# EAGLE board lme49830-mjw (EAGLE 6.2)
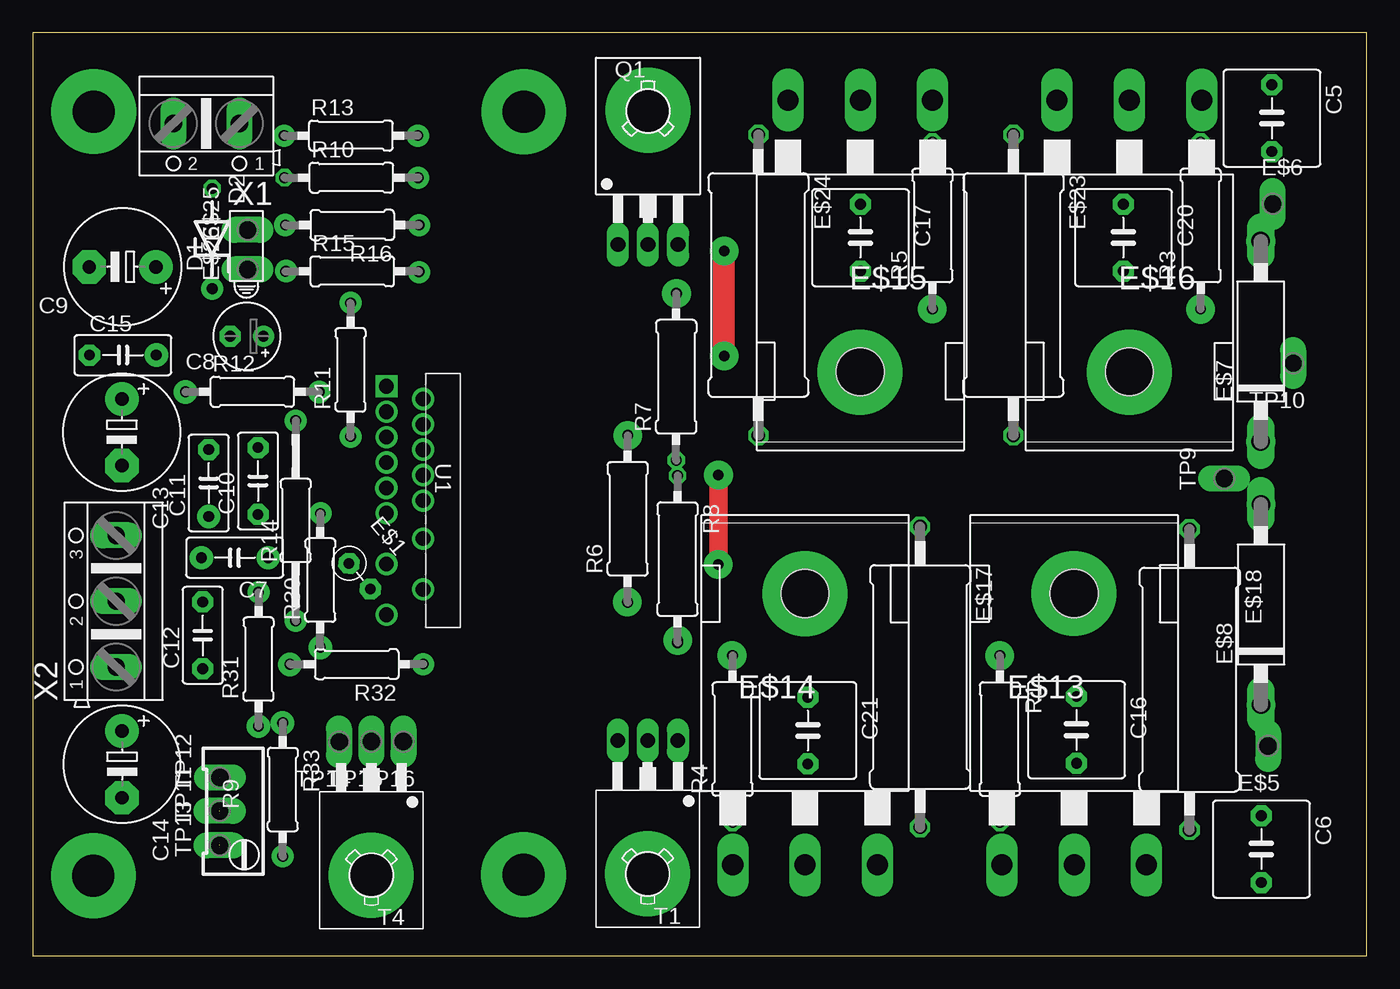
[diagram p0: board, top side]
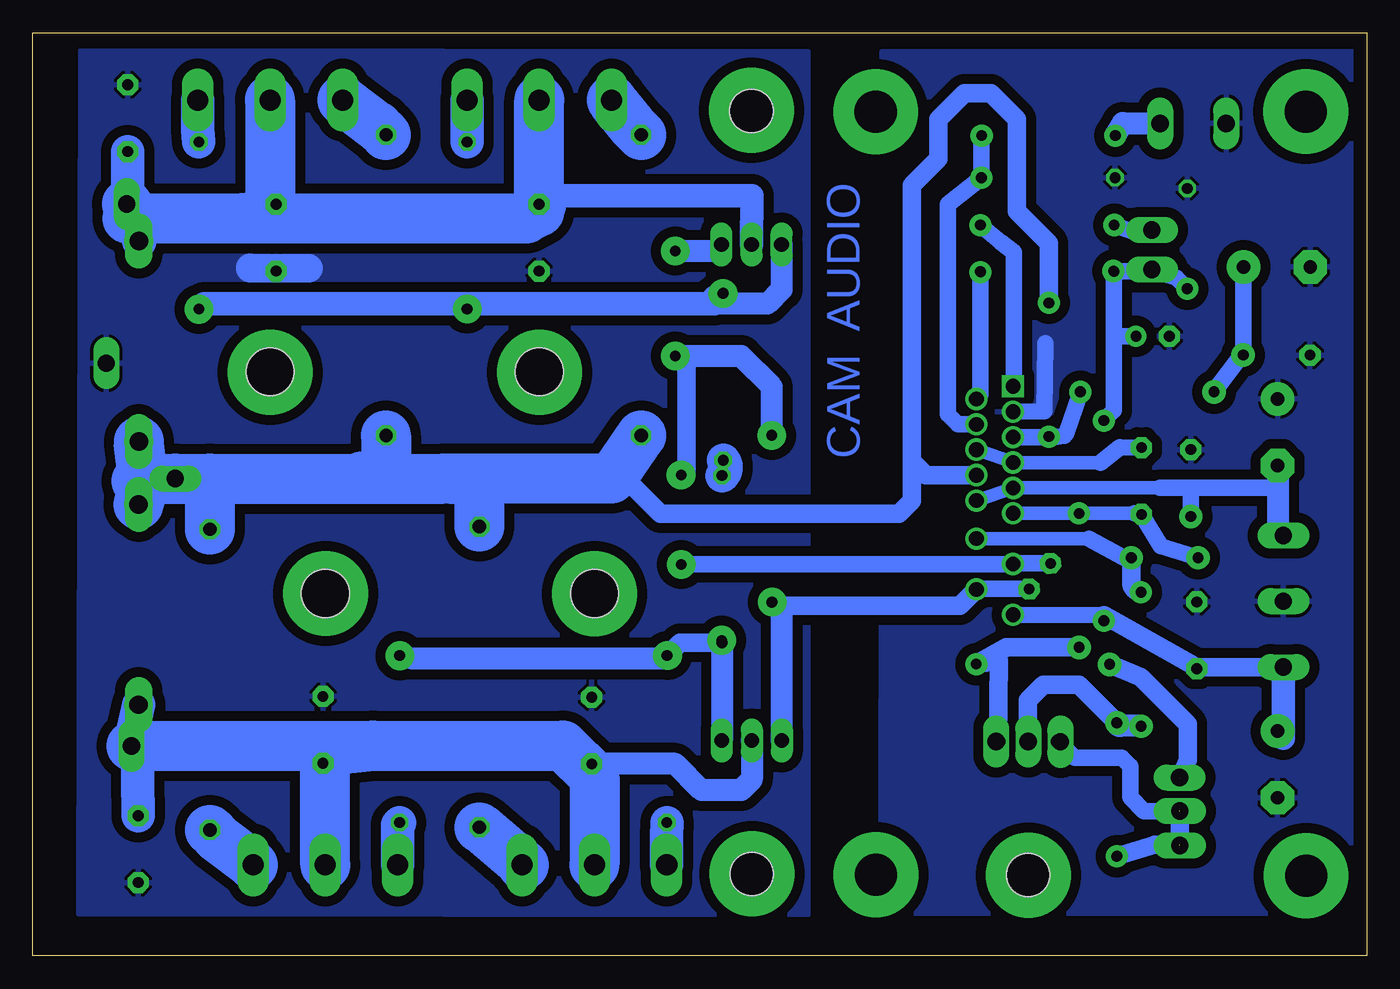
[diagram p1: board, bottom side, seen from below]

Size 101.46 x 70.17 mm. Coordinates in mm from the lower left corner, seen from the top.
Outline: 0,0 101.46,0 101.46,70.17 0,70.17 0,0
Copper layers (1*16): Top 0.035mm / dielectric 1.5mm / Bottom 0.035mm
Design rules: minimum track width 10mil, minimum drill 24mil, track to track 30mil, track to pad 30mil, pad to pad 30mil, via to via 30mil, smd to smd 30mil, copper to edge 40mil, drill to drill 8mil, minimum pad ring 10mil, minimum via ring 8mil, stop-mask expansion 4mil, vias tented up to drill 0mil, thermal gap 10mil
vRestrict: area 32.5,1.9 to 43.5,68.9

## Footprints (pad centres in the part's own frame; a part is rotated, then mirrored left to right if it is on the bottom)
C5B7.2 = drill 0.813 pad 1.6 octagon: 1 -2.54,0; 2 2.54,0
C5B3 = drill 0.813 pad 1.6 octagon: 1 -2.54,0; 2 2.54,0
E2,5-5 = drill 0.813 pad 1.6: + -1.27,0 | drill 0.813 pad 1.6 octagon: - 1.27,0
E5-8,5 = drill 1.016 pad 2.54: + -2.54,0 | drill 1.016 pad 2.54 octagon: - 2.54,0
ZDIO-7.5 = drill 0.813 octagon: A 3.81,0; C -3.81,0
HLMP6 = drill 0.813 long: A -1.27,0; K 1.27,0
RS-2,5 = drill 0.813 pad 1.6 octagon: 1 -1.27,0; 2 1.27,0
P1-13Y = drill 1.321 pad 1.905 long: TP 0,0
C1702E15 = drill 1.397 long: A 7.62,0; C -7.62,0
TO-247AD-H = drill 1.6 long: D 0,-20.65; G -5.5,-20.65; S 5.5,-20.65 | hole 3.65: 0,0
P0817/22 = drill 1.016 octagon: 1 -11.43,0; 2 11.43,0
TO126 = drill 1.118 long: 1 -2.286,-5.08; 2 0,-5.08; 3 2.286,-5.08 | hole 3.302: 0,5.08
0309/12 = drill 0.813 octagon: 1 -6.35,0; 2 6.35,0
RTRIM64W = drill 0.61: 1 1.27,-2.54; 2 1.27,0; 3 1.27,2.54
0207/10 = drill 0.813 octagon: 1 -5.08,0; 2 5.08,0
0207/15 = drill 0.813 octagon: 1 -7.62,0; 2 7.62,0
TB15A = drill 1.118 square: 1 -17.374,-8.611 | drill 1.118: 2 -16.408,-5.817; 3 -15.443,-8.611; 4 -14.478,-5.817; 5 -13.513,-8.611; 6 -12.548,-5.817; 7 -11.582,-8.611; 8 -10.617,-5.817; 9 -9.652,-8.611; 10 -8.687,-5.817; 11 -7.722,-8.611; 12 -5.791,-5.817; 13 -3.861,-8.611; 14 -1.93,-5.817; 15 0,-8.611
AK500/2 = drill 1.321 long: 1 -2.515,0; 2 2.515,0
AK500/3 = drill 1.321 long: 1 -5.004,0; 2 0,0; 3 5.004,0

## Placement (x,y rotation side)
C5  [C5B7.2]  94.25,63.68 270 top
C6  [C5B7.2]  93.45,8.1 270 top
C7  22p  [C5B3]  15.36,30.26 180 top
C8  47u  [E2,5-5]  16.28,47.1 180 top
C9  220u  [E5-8,5]  6.83,52.38 180 top
C10  22p  [C5B3]  17.13,36.09 90 top
C11  100n  [C5B3]  13.38,35.94 90 top
C12  100n  [C5B3]  12.92,24.36 90 top
C13  100u  [E5-8,5]  6.77,39.8 270 top
C14  100u  [E5-8,5]  6.78,14.55 270 top
C15  100n  [C5B3]  6.85,45.67 0 top
C16  [C5B7.2]  79.39,17.17 270 top
C17  [C5B7.2]  62.95,54.6 270 top
C20  [C5B7.2]  82.95,54.6 270 top
C21  [C5B7.2]  58.95,17.12 270 top
D1  5v1  [ZDIO-7.5]  13.64,54.53 90 top
D2  HLMP6  [HLMP6]  16.25,53.71 90 top
E$1  [RS-2,5]  24.86,28.86 310 top
E$5  [P1-13Y]  93.97,15.95 180 top
E$6  [P1-13Y]  94.32,57.17 0 top
E$7  [C1702E15]  93.4,46.71 90 top
E$8  [C1702E15]  93.42,26.7 90 top
E$13  MJL4281  [TO-247AD-H]  79.21,27.55 0 top
E$14  MJL4281  [TO-247AD-H]  58.74,27.55 0 top
E$15  MJL4302  [TO-247AD-H]  62.94,44.4 180 top
E$16  MJL4302  [TO-247AD-H]  83.41,44.4 180 top
E$17  0,3  [P0817/22]  67.49,21.19 270 top
E$18  0,3  [P0817/22]  87.99,20.99 270 top
E$23  0,3  [P0817/22]  74.59,50.99 270 top
E$24  0,3  [P0817/22]  55.19,50.99 270 top
E$25  [P1-13Y]  16.34,55.19 90 top
E$26  [P1-13Y]  16.34,52.19 90 top
Q1  BD140  [TO126]  46.79,59.15 0 top
R1  10  [0309/12]  73.56,16.47 270 top
R3  10  [0309/12]  88.83,55.53 90 top
R4  10  [0309/12]  53.23,16.47 90 top
R5  10  [0309/12]  68.43,55.53 90 top
R6  2k2  [0309/12]  45.25,33.22 90 top
R7  100  [0309/12]  48.94,44.02 90 top
R8  100  [0309/12]  49.04,30.15 270 top
R9  200  [RTRIM64W]  15.49,10.99 180 top
R10  6k8  [0207/10]  24.23,59.16 0 top
R11  6k8  [0207/10]  24.17,44.55 90 top
R12  243  [0207/10]  16.7,42.88 0 top
R13  243  [0207/10]  24.2,62.36 0 top
R14  22k  [0207/15]  20,33.08 90 top
R15  33k  [0207/10]  24.3,52.04 0 top
R16  470  [0207/10]  24.3,55.56 180 top
R30  10  [0207/10]  21.87,28.55 90 top
R31  0  [0207/10]  17.17,22.55 90 top
R32  330  [0207/10]  24.63,22.17 180 top
R33  1k2  [0207/10]  19.01,12.63 270 top
T1  BD139  [TO126]  46.77,11.29 180 top
T4  bd139  [TO126]  25.75,11.21 180 top
TP9  PTR1PAD1-13Y  [P1-13Y]  90.63,36.28 90 top
TP10  PTR1PAD1-13Y  [P1-13Y]  95.88,45.05 180 top
TP11  TPPAD1-13Y  [P1-13Y]  14.21,11.01 90 top
TP12  TPPAD1-13Y  [P1-13Y]  14.22,13.54 90 top
TP13  TPPAD1-13Y  [P1-13Y]  14.21,8.39 90 top
TP14  TPPAD1-13Y  [P1-13Y]  23.3,16.27 180 top
TP15  TPPAD1-13Y  [P1-13Y]  25.74,16.28 180 top
TP16  TPPAD1-13Y  [P1-13Y]  28.19,16.28 180 top
U1  LME49810  [TB15A]  35.51,25.92 270 top
X1  [AK500/2]  13.2,63.28 180 top
X2  [AK500/3]  6.34,26.95 90 top

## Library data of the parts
C5-C7 C10-C12 C15-C17 C20 C21 = capacitor-wima
C8 E$17 E$18 E$23 E$24 R1 R3-R16 R30-R33 = rcl
C9 C13 C14 = resistor
D1 E$7 E$8 = diode
D2 = display-hp; MF: AGILENT TECHNOLOGIES; MPN: HLMP-6500; OC_FARNELL: 1652490; OC_NEWARK: 40K0088
E$1 = discrete
E$5 E$6 E$25 E$26 TP9-TP16 = testpad
E$13-E$16 = transistor-power
Q1 = transistor-pnp
T1 T4 = transistor-neu-to92
U1 = lme49830
X1 X2 = con-ptr500

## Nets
GND4: C5.1 C6.2 C16.1 C17.2 C20.2 C21.1 TP10.TP
GND6: C8.- C9.- C11.2 C12.2 C13.+ C14.- C15.1 D1.A R10.1 U1.3 X1.2 X2.2
N$1: E$15.S E$24.1
N$2: E$16.S E$23.1
N$3: E$14.S E$17.2
N$4: E$13.S E$18.2
N$5: R1.1 R4.2 R8.2 T1.1
N$6: Q1.1 R3.1 R5.1 R7.2
N$7: C6.1 C16.2 C21.2 E$5.TP E$8.C E$13.D E$14.D T1.2
N$8: C5.2 C17.1 C20.1 E$6.TP E$7.A E$15.D E$16.D Q1.2
N$9: E$16.G R3.2
N$11: E$14.G R4.1
N$12: E$15.G R5.2
N$13: E$1.2 R6.1 T1.3 U1.14
N$14: E$1.1 Q1.3 R6.2 U1.13
N$15: E$7.C E$8.A E$17.1 E$18.1 E$23.2 E$24.2 R11.2 TP9.TP U1.8
N$16: R11.1 R12.2 U1.5
N$17: R10.2 R13.2 U1.4
N$18: C9.+ C15.2 R12.1
N$19: R13.1 X1.1
N$20: C8.+ D1.C D2.A R14.2 R15.1
N$21: C10.2 U1.6
N$22: D2.K R16.2
N$23: R16.1 U1.1
N$24: R15.2 U1.2
S$10: E$13.G R1.2
S$40: R7.1 R8.1
S$51: C7.2 C10.1 R30.2 U1.11
S$52: C7.1 R31.2 U1.12
S$102: R31.1 R33.1 T4.2
S$103: R30.1 R32.1 T4.1
S$104: R9.1 R32.2 TP12.TP
S$105: R9.2 R9.3 R33.2 T4.3 TP11.TP TP13.TP
VCC1: C12.1 C14.+ R14.1 U1.15 X2.1
VEE1: C11.1 C13.- U1.10 X2.3

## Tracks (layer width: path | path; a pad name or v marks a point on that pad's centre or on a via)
GND4
  Bottom 2.184: 80.48,52.28 84.92,52.28 84.92,52.29
  pour Bottom: 42.49,68.72 97.83,68.8 97.96,3.19 42.48,3.1
GND6  (via drill 0.6 pad 1.68)
  Bottom 1.27: 26.85,41.36 24.51,41.38 24.45,46.57
  other vias: 26.9,41.36
  pour Bottom: 36.86,68.73 36.96,3.17 0.94,3.22 1,68.73
N$1
  Bottom 3.81: E$15.S 55.82,63.05 E$24.1
N$2
  Bottom 3.81: E$16.S 75.22,63.05 E$23.1
N$3
  Bottom 3.81: E$14.S 64.13,6.9 E$17.2
N$4
  Bottom 3.81: E$13.S 87.33,8.9 E$18.2
N$5
  Bottom 1.422: R8.2 52.25,23.8 R4.2 | T1.1 49.04,16.04
  Bottom 1.676: R4.2 53.46,22.59 72.59,22.59 R1.1 | R8.2 49.04,16.39 T1.1
N$6
  Bottom 1.676: Q1.1 44.51,50.67 45.59,49.59 49.59,49.59
  Bottom 1.778: R3.1 88.42,49.59 68.43,49.59 | 68.43,49.59 49.59,49.59 49.59,50.07 R7.2 | R5.1 68.43,49.59
N$7
  Bottom 1.27: 58.67,13.67 58.74,13.59
  Bottom 1.422: C21.2 58.95,13.95 58.67,13.67
  Bottom 1.676: C16.2 82.74,16.06 arc-90 79.21,15.59 | T1.2 46.77,13.41 47.59,12.59 50.59,12.59 52.59,14.59 58.94,14.59 C21.2
  Bottom 2.54: E$8.C 94.13,15.97 E$5.TP 93.54,16.23 C6.1
  Bottom 3.81: E$5.TP 75.59,15.97 | 75.59,15.97 61.13,15.97 58.74,13.59 E$14.D | E$13.D 79.21,15.59 75.59,15.97
N$8
  Bottom 1.676: C17.1 61.95,56.45 arc-90 62.09,57.79 | C20.1 82.95,55.23 82.59,55.59 82.59,56.07
  Bottom 1.778: Q1.2 46.75,57.79 62.09,57.79 62.94,56.59
  Bottom 2.54: E$7.A 93.34,54.3 E$6.TP | C5.2 94.25,56.07
  Bottom 3.81: E$6.TP 93.59,56.07 | 94.25,56.07 93.59,56.07 | 93.59,56.07 85.59,56.07 | 85.59,56.07 82.59,56.07 63.94,56.07 62.94,56.59 E$15.D | E$16.D 83.41,56.25 85.59,56.07
N$9
  Bottom 2.54: E$16.G 88.91,62.8 R3.2
N$11
  Bottom 2.54: E$14.G 53.24,9.13 R4.1
N$12
  Bottom 2.54: E$15.G R5.2
N$13
  Bottom 1.27: E$1.2 29.69,27.88 U1.14
  Bottom 1.422: U1.14 30.95,26.59 44.97,26.59 R6.1
  Bottom 1.676: T1.3 44.49,26.11 R6.1
N$14  (via drill 0.6, 0.8 pad 2.18)
  Top 1.422: v52.14,29.76 v52.15,36.56
  Top 1.676: v52.59,45.59 v52.59,53.59
  Bottom 1.27: v52.14,29.76 43.42,29.78 40.36,29.78 26.99,29.77 U1.13 26.89,29.83 E$1.1
  Bottom 1.422: v52.15,36.56 arc-90 51.74,36.96 51.74,45.59
  Bottom 1.676: R6.2 45.25,43.25 47.59,45.59 51.74,45.59 v52.59,45.59 | v52.59,53.59 49.56,53.59 Q1.3
N$15
  Bottom 1.422: U1.8 33.54,36.54 34.59,37.59 | 34.59,37.59 34.59,58.59 32.59,60.59 32.59,63.59 30.59,65.59 28.59,65.59 26.59,63.59 26.59,56.59 24.17,54.17 R11.2 | 34.59,37.59 34.59,34.59 35.59,33.59 53.73,33.59 57.04,36.9
  Bottom 3.81: 87.99,36.28 TP9.TP 92.84,36.28 | 87.99,36.28 76.59,36.28 | 76.59,36.28 70.19,36.28 | 76.59,36.28 76.44,36.44 74.59,36.44 E$23.2 | 70.19,36.28 67.49,36.08 E$17.1 | 93.59,36.08 93.39,36.28 93.06,36.28 | 93.06,36.28 E$7.C | E$8.A 92.84,36.28 | E$18.1 87.99,36.28 | 93.06,36.28 92.84,36.28 | E$24.2 57.04,36.9 57.47,36.28 70.19,36.28
N$16
  Bottom 1.27: U1.5 24.2,39.43 R11.1 23.55,39.47 22.99,39.53 22.82,39.72 21.81,42.68 R12.2
N$17  (via drill 0.8 pad 1.68)
  Bottom 1.27: U1.4 31.07,40.4 31.85,41.17 31.85,57.12 R10.2 29.31,62.33 v29.29,62.35 R13.2
N$18
  Bottom 1.27: C9.+ 9.37,46 9.39,45.85 | 9.39,45.85 C15.2 | R12.1 9.39,45.85
N$19
  Bottom 1.676: R13.1 18.56,63.31 X1.1
N$20
  Bottom 1.27: 17.53,47.08 C8.+ 19.1,47.11 19.22,46.99 | 16.12,52.04 R15.1 19.22,46.99 | 16.12,52.04 14.48,51.56 D1.C | D2.A 16.42,52.15 16.12,52.04 | 19.22,46.99 19.22,41.48 R14.2
N$21
  Bottom 1.016: U1.6 26.75,37.47 20.25,37.47
  Bottom 1.27: 20.25,37.47 18.77,38.65 C10.2
N$22  (via drill 0.8 pad 1.68)
  Bottom 1.27: D2.K 17.54,54.98 R16.2 v19.21,55.56
N$23
  Bottom 1.27: R16.1 27.84,54.26 26.85,53.47 26.85,43.34 U1.1
N$24  (via drill 0.8 pad 1.68)
  Bottom 1.27: R15.2 v29.38,51.98 29.38,42.64 U1.2
N$25  (via drill 3.2 pad 6.45)
  other vias: 37.35,64.17
N$26  (via drill 3.2 pad 6.45)
  other vias: 46.78,64.29
N$27  (via drill 0.6 pad 1.68)
  other vias: 29.69,42.31
N$28  (via drill 0.6 pad 1.68)
  other vias: 29.69,40.4
N$29  (via drill 0.6 pad 1.68)
  other vias: 29.7,38.49
N$30  (via drill 0.6 pad 1.68)
  other vias: 29.69,36.55
N$31  (via drill 0.6 pad 1.68)
  other vias: 29.68,34.6
N$32  (via drill 0.6 pad 1.68)
  other vias: 29.69,31.69
N$33  (via drill 0.6 pad 1.68)
  other vias: 29.7,27.86
N$34  (via drill 0.6 pad 1.68)
  other vias: 26.9,25.91
N$35  (via drill 0.6 pad 1.68)
  other vias: 26.9,29.77
N$36  (via drill 0.6 pad 1.68)
  other vias: 26.91,33.63
N$37  (via drill 0.6 pad 1.68)
  other vias: 26.89,35.55
N$38  (via drill 0.6 pad 1.68)
  other vias: 26.91,37.48
N$43  (via drill 0.6 pad 1.68)
  other vias: 26.9,39.43
N$48  (via drill 0.6 pad 1.68)
  other vias: 26.91,43.29
N$49  (via drill 0.8 pad 1.68)
  other vias: 29.38,55.55
N$55  (via drill 0.8 pad 1.68)
  other vias: 24.16,39.46
N$56  (via drill 0.8 pad 1.68)
  other vias: 29.32,59.16
N$58  (via drill 0.8 pad 1.68)
  other vias: 19.12,62.35
N$104  (via drill 0.8 pad 1.68)
  other vias: 24.16,49.64
N$105  (via drill 0.8 pad 1.68)
  other vias: 19.25,52.06
N$106  (via drill 0.8 pad 1.68)
  other vias: 13.65,50.7
N$107  (via drill 0.8 pad 1.68)
  other vias: 19.99,40.69
N$108  (via drill 0.8 pad 1.68)
  other vias: 21.78,42.86
N$109  (via drill 0.8 pad 1.68)
  other vias: 19.99,25.46
N$110  (via drill 3.2 pad 6.45)
  other vias: 4.6,6.06
N$111  (via drill 3.2 pad 6.45)
  other vias: 4.63,64.19
N$112  (via drill 0.8 pad 1.78)
  other vias: 11.62,42.87
N$113  (via drill 0.8 pad 1.78)
  other vias: 9.4,45.67
N$114  (via drill 0.8 pad 1.78)
  other vias: 12.82,30.26
N$115  (via drill 0.8 pad 1.78)
  other vias: 13.38,33.4
N$116  (via drill 0.8 pad 1.78)
  other vias: 21.88,23.43
N$117  (via drill 0.8 pad 1.78)
  other vias: 18.99,17.69
N$118  (via drill 0.8 pad 1.78)
  other vias: 17.16,17.44
N$119  (via drill 0.8 pad 1.78)
  other vias: 19.55,22.15
S$10
  Bottom 2.54: E$13.G 73.71,9.97 R1.2
S$11  (via drill 1 pad 1.68)
  other vias: 58.74,6.9
S$12  (via drill 1 pad 1.68)
  other vias: 64.24,6.9
S$13  (via drill 1 pad 1.68)
  other vias: 53.24,6.9
S$14  (via drill 1 pad 1.68)
  other vias: 73.72,6.89
S$15  (via drill 1 pad 1.68)
  other vias: 84.71,6.91
S$16  (via drill 1 pad 1.68)
  other vias: 79.22,6.89
S$23  (via drill 0.8 pad 1.68)
  other vias: 62.94,65.02
S$24  (via drill 0.8 pad 1.68)
  other vias: 68.44,65.03
S$28  (via drill 0.8 pad 1.68)
  other vias: 57.45,65.02
S$32  (via drill 0.8 pad 1.68)
  other vias: 83.42,65.06
S$34  (via drill 0.8 pad 1.68)
  other vias: 88.91,65.05
S$36  (via drill 0.8 pad 1.68)
  other vias: 77.91,65.06
S$40
  Bottom 2.54: R8.1 48.98,36.54 arc-90 R7.1
S$45  (via drill 3.2 pad 6.45)
  other vias: 58.74,27.51
S$46  (via drill 3.2 pad 6.45)
  other vias: 79.2,27.54
S$49  (via drill 3.2 pad 6.45)
  other vias: 83.4,44.37
S$50  (via drill 3.2 pad 6.45)
  other vias: 62.92,44.37
S$51
  Bottom 0.406: R30.2 23.59,33.63 23.59,33.64
  Bottom 1.016: U1.11 23.59,33.64 17.67,33.64
  Bottom 1.27: 17.67,33.64 17.27,33.55 C10.1 15.66,31.14 C7.2
S$52  (via drill 0.8 pad 1.78)
  Bottom 1.016: U1.12 21.14,31.71
  Bottom 1.27: 29.73,31.67 U1.12 | 21.14,31.71 18.46,30.25 C7.1
  Bottom 1.422: C7.1 17.9,28.36 arc-90 R31.2
  other vias: 17.9,30.26
S$54  (via drill 3.2 pad 6.45)
  other vias: 25.74,6.12
S$57  (via drill 3.2 pad 6.45)
  other vias: 37.33,6.14
S$58  (via drill 3.2 pad 6.45)
  other vias: 46.75,6.22
S$59  (via drill 0.8 pad 1.68)
  other vias: 16.34,55.19
S$60  (via drill 0.8 pad 1.68)
  other vias: 16.34,52.19
S$61  (via drill 0.8 pad 1.78)
  other vias: 4.63,64.19
S$62  (via drill 0.8 pad 1.78)
  other vias: 37.34,64.17
S$63  (via drill 0.8 pad 1.78)
  other vias: 37.36,6.14
S$64  (via drill 0.8 pad 1.78)
  other vias: 4.6,6.06
S$81  (via drill 0.8 pad 1.78)
  other vias: 14.26,10.95
S$100  (via drill 0.8 pad 1.78)
  other vias: 14.23,13.55
S$101  (via drill 0.8 pad 1.78)
  other vias: 14.19,8.44
S$102
  Bottom 1.422: R33.1 21.89,20.59 24.59,20.59 25.75,19.43 T4.2
  Bottom 1.676: R31.1 18.77,17.47 arc90 R33.1
S$103
  Bottom 1.422: R30.1 27.41,23.47 R32.1 27.99,22.44 T4.1
S$104  (1 unrouted)
  Bottom 1.422: R32.2 17.17,21.17 13.59,17.59 13.59,14.9 R9.1
S$105  (2 unrouted)
  Bottom 1.27: T4.3 22.21,15.03 18.61,15.03 17.98,14.4 17.98,12.03 16.94,10.99 R9.2
  Bottom 1.422: R33.2 16.12,8.45 R9.3 R9.2
S$106  (via drill 0.8 pad 2.18)
  other vias: 88.82,49.16
S$107  (via drill 0.8 pad 2.18)
  other vias: 68.42,49.17
S$108  (via drill 0.8 pad 2.18)
  other vias: 48.97,50.36
S$109  (via drill 0.8 pad 2.18)
  other vias: 49.05,23.98
S$110  (via drill 0.8 pad 2.18)
  other vias: 53.19,22.83
S$111  (via drill 0.8 pad 2.18)
  other vias: 45.22,26.88
S$112  (via drill 0.8 pad 2.18)
  other vias: 45.25,39.55
S$113  (via drill 0.8 pad 2.18)
  other vias: 52.15,36.56
S$114  (via drill 0.8 pad 2.18)
  other vias: 52.14,29.75
S$115  (via drill 0.8 pad 2.18)
  other vias: 73.55,22.81
S$116  (via drill 0.8 pad 1.68)
  other vias: 21.87,33.64
S$117  (via drill 0.8 pad 1.68)
  other vias: 17.17,27.63
S$118  (via drill 0.8 pad 1.68)
  other vias: 19,7.56
S$119  (via drill 0.8 pad 1.68)
  other vias: 29.7,22.16
S$120  (via drill 0.8 pad 1.68)
  other vias: 25.76,6.09
S$121  (via drill 0.8 pad 1.68)
  other vias: 46.78,6.18
S$122  (via drill 0.8 pad 1.68)
  other vias: 46.78,64.28
S$123  (via drill 0.8 pad 2.18)
  other vias: 58.74,27.52
S$127  (via drill 0.8 pad 2.18)
  other vias: 62.93,44.4
S$128  (via drill 0.8 pad 2.18)
  other vias: 83.41,44.4
S$129  (via drill 0.8 pad 2.18)
  other vias: 79.19,27.54
S$134  (via drill 0.8 pad 2.18)
  other vias: 93.43,19.07
S$135  (via drill 0.8 pad 2.18)
  other vias: 93.42,34.32
S$136  (via drill 0.8 pad 2.18)
  other vias: 93.41,39.08
S$137  (via drill 0.8 pad 2.18)
  other vias: 93.4,54.33
VCC1
  Bottom 0.406: R14.1 19.56,25.46 19.56,25.64
  Bottom 1.27: 26.75,25.77 U1.15 | C14.+ 6.79,16.99 | 6.79,16.99 6.79,17.25 | U1.15 20,25.89 | 26.89,25.91 U1.15 | 27.04,25.77 U1.15 | 6.8,16.99 6.79,16.99
  Bottom 1.422: 20,25.89 19.56,25.64 12.89,21.89 | 12.89,21.89 12.82,21.82 C12.1 | 12.89,21.89 12.95,21.95 X2.1
  Bottom 1.778: X2.1 6.34,16.53 C14.+
VEE1
  Bottom 1.016: U1.10 26.85,35.57 15.75,35.57
  Bottom 1.27: 29.73,34.57 U1.10 | 15.75,35.57 13.33,35.57 | 13.33,35.57 6.88,35.57 6.77,35.68 | C11.1 13.38,35.52 13.33,35.57
  Bottom 1.676: C13.- 6.77,35.68 6.77,32.38 X2.3

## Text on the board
Bottom: AUDIO | CAM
